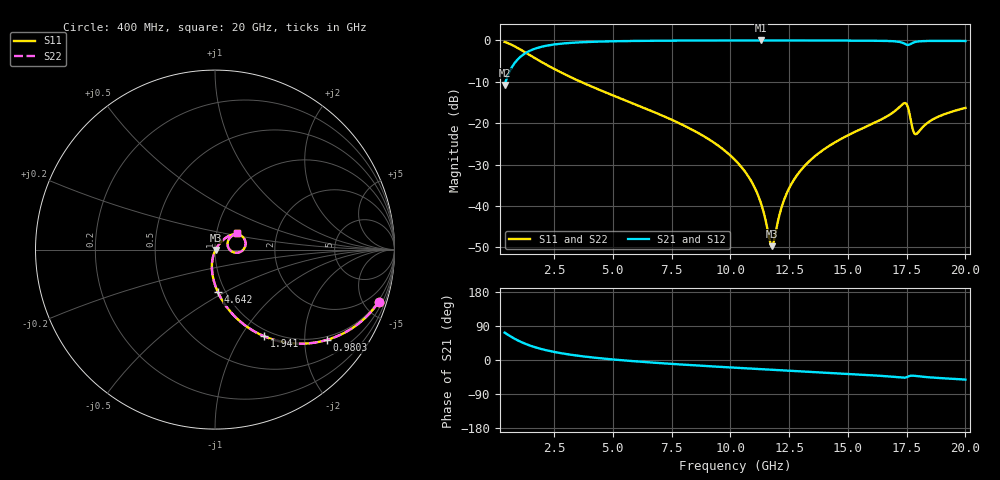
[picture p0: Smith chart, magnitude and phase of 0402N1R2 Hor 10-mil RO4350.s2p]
# GHz S MA R 50
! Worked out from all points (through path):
!   1960 points, 400 MHz to 20 GHz, reference 50 ohm
!   highest |S21| = -0.03 dB at 11.31 GHz (marker M1); lowest = -10.8 dB at 400 MHz (marker M2)
!   group delay of S21, straight-line fit = 12.7 ps
!   lowest |S11| = -49.7 dB at 11.77 GHz (marker M3), VSWR 1.01, Z = 50.3 - j0.149 ohm
!   |S11| at or under -10 dB: 3.636 GHz to end of sweep
!   |S22| runs from -49.7 to -0.4 dB; largest |S21 - S12| = 0
!   S11 on the Smith chart (normalised r, x): 400 MHz: 0.91, -6.29; 980.3 MHz: 0.91, -2.55; 1.941 GHz: 0.91, -1.27; 4.642 GHz: 0.92, -0.47; 20 GHz: 1.26, +0.23
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0.4  0.9571 -17.7  0.2895 72.3  0.2895 72.3  0.9571 -17.7
0.9802961  0.8016 -38.9  0.5973 51.1  0.5973 51.1  0.8016 -38.9
1.940786  0.5538 -60.6  0.8315 29.3  0.8315 29.3  0.5538 -60.6
3.671669  0.3129 -79.6  0.9479 10.1  0.9479 10.1  0.3129 -79.6
4.642164  0.2387 -86.0  0.969 3.5  0.969 3.5  0.2387 -86.0
6.943338  0.1294 -96.8  0.9889 -7.9  0.9889 -7.9  0.1294 -96.8
8.914344  0.06852 -103.4  0.9945 -15.7  0.9945 -15.7  0.06852 -103.4
10.205  0.03591 -105.6  0.9959 -20.4  0.9959 -20.4  0.03591 -105.6
10.85533  0.02077 -104.0  0.9962 -22.6  0.9962 -22.6  0.02077 -104.0
11.30556  0.01079 -97.0  0.9963 -24.2  0.9963 -24.2  0.01079 -97.0
11.7658  0.003279 -26.9  0.9962 -25.8  0.9962 -25.8  0.003279 -26.9
11.85584  0.003813 4.1  0.9962 -26.1  0.9962 -26.1  0.003813 4.1
12.17601  0.009543 42.2  0.9961 -27.1  0.9961 -27.1  0.009543 42.2
12.45615  0.01541 49.1  0.9959 -28.1  0.9959 -28.1  0.01541 49.1
13.46667  0.03707 52.8  0.9951 -31.5  0.9951 -31.5  0.03707 52.8
16.73834  0.1244 41.9  0.9812 -43.3  0.9812 -43.3  0.1244 41.9
17.4487  0.1745 13.1  0.8992 -46.3  0.8992 -46.3  0.1745 13.1
17.56876  0.1515 -2.5  0.8802 -43.6  0.8802 -43.6  0.1515 -2.5
17.78887  0.0797 1.3  0.9393 -41.4  0.9393 -41.4  0.0797 1.3
17.90893  0.074 18.0  0.9605 -42.3  0.9605 -42.3  0.074 18.0
18.68933  0.1141 38.8  0.9839 -46.7  0.9839 -46.7  0.1141 38.8
20  0.153 36.2  0.9817 -51.6  0.9817 -51.6  0.153 36.2
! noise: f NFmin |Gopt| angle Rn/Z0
0.4  0.001328  0.8187  5.238  0.001531
2.571  0.005089  0.6818  7.825  0.003083
4.752  0.008085  0.6383  11.93  0.004173
6.933  0.01078  0.6117  16.24  0.005054
9.104  0.01331  0.5937  20.55  0.00583
11.29  0.01579  0.5819  24.83  0.006583
13.47  0.01843  0.5776  29.04  0.007462
15.64  0.02281  0.6018  33.25  0.009755
17.82  0.0782  0.8489  38.36  0.09835
20  0.02769  0.5929  41.57  0.011
